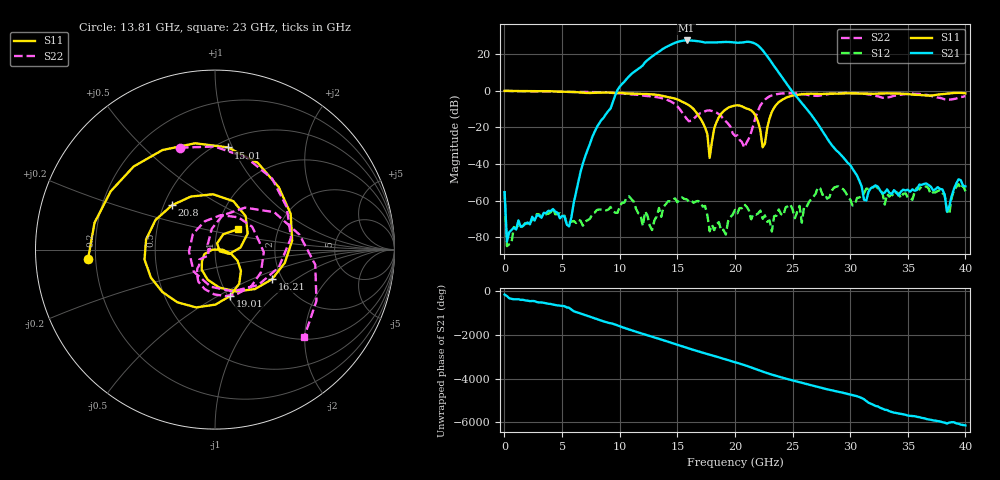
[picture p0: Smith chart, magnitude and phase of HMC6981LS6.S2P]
! Hittite Microwave Corporation
! 2 Elizabeth Drive
! Chelmsford, MA 01824
! http://www.hittite.com
! Tel: 978-250-3343
! Fax: 978-250-3373
! Device:  HMC6981LS6
! Description: GaAs pHEMT MMIC 2 WATT POWER AMPLIFIER, 15 - 20 GHz
! Package:  LS6
! Ports:  Pad 1 = Vdd3
!  Pad 2 = Vdd2
!  Pad 3 = Vdd1
!  Pad 4 = Vgg1
!  Pad 5 = GND
!  Pad 6 = RFIN (RF Port 1)
!  Pad 7 = GND
!  Pad 8 = N/C
!  Pad 9 = Vgg2
!  Pad 10 = Vdd5
!  Pad 11 = Vref
!  Pad 12 = Vdet
!  Pad 13 = GND
!  Pad 14 = RFOUT (RF Port 2)
!  Pad 15 = GND
!  Pad 16 = Vdd4
!  Exposed Ground Paddle = GND
! Conditions:  All Vdd = 6.0 Volts
!  Vgg1 or Vgg2 voltage adjusted to obtain quiescent Idd = 1100 mA
!  Ambient temperature approximately +25 deg C
! Hardware:  The device was measured using:
!  LM, EVAL 090-01115-00 Rev B
!  PCB, EVAL 600-00649-00 Rev 1
!  AD, EVAL 115-00651-00 Rev 1
! Misc:  Validation SN7
! Note:  Hittite supplies this file as a sample of data as measured at the Evaluation PCB's coaxial connectors.
!  Your particular measurements for this product may vary from device to device.
!  Hittite reserves the right to change this data at any time.
# GHZ S DB R 50
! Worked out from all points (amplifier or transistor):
!   201 points, 10 MHz to 40 GHz, reference 50 ohm
!   highest |S21| = 27.2 dB at 15.81 GHz (marker M1)
!   |S21| within 3 dB of that: 14.21 GHz to 22.05 GHz (7.837 GHz wide, 43.2 % of centre)
!   unconditionally stable (mu >= 1): start of sweep to end of sweep
!   at 6.608 GHz: K = 10659.95, MAG = -29.9 dB, |S12| = -70.9 dB
!   at 20 GHz: K = 37.20, MAG = 26.8 dB, |S12| = -65.0 dB
!   at 40 GHz: K = 16637.74, MAG = -43.9 dB, |S12| = -54.9 dB
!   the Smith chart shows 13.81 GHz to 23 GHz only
!   S11 on the Smith chart (normalised r, x): 13.81 GHz: 0.17, -0.04; 15.01 GHz: 0.57, +0.96; 16.21 GHz: 1.77, -0.67; 19.01 GHz: 1.03, -0.57; 20.8 GHz: 0.55, +0.31; 23 GHz: 1.26, +0.30
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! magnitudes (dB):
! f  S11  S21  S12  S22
! 10 MHz  -0.2  -55.4  -54.7  -0.2
! 209.9 MHz  -0.2  -82.2  -84.7  -0.2
! 5.609 GHz  -0.7  -74.0  -71.9  -0.8
! 6.808 GHz  -1.2  -39.7  -73.6  -0.8
! 10.01 GHz  -1.3  2.1  -63.0  -1.5
! 12.81 GHz  -2.1  18.5  -75.9  -3.3
! 13.41 GHz  -2.5  21.1  -63.9  -3.8
! 13.81 GHz  -3.0  22.9  -63.2  -4.4
! 15.01 GHz  -4.8  26.5  -60.8  -8.7
! 15.81 GHz  -7.3  27.2  -59.2  -15.4
! 16.21 GHz  -8.9  27.2  -59.9  -16.4
! 17.81 GHz  -36.7  26.2  -76.6  -10.8
! 19.01 GHz  -11.3  26.4  -75.8  -15.6
! 20.2 GHz  -8.0  26.0  -66.8  -24.4
! 20.8 GHz  -9.3  26.3  -62.0  -31.1
! 22.4 GHz  -30.9  21.9  -69.8  -6.4
! 23 GHz  -15.2  16.9  -70.7  -3.2
! 26.8 GHz  -1.8  -14.7  -57.8  -2.8
! 31.2 GHz  -1.7  -59.5  -55.9  -1.8
! 33.4 GHz  -1.6  -55.6  -57.8  -3.7
! 38.4 GHz  -1.8  -65.9  -65.6  -4.8
! 40 GHz  -1.5  -52.2  -54.9  -3.0
